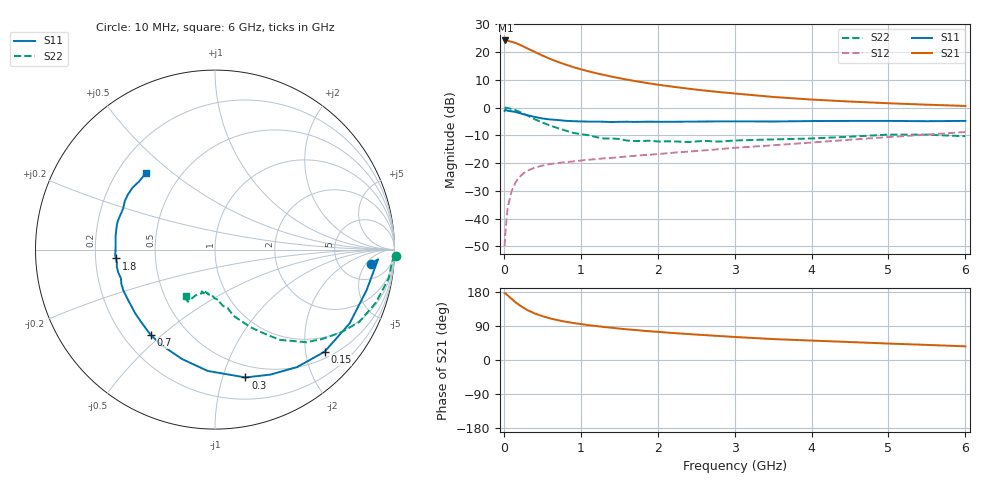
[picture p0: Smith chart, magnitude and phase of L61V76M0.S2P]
!  INFINEON TECHNOLOGIES Small Signal Semiconductors
! BFR380L3 , Si-NPN RF-Transistor in TSLP-3-1
!  Vce=1.75 V,  Ic=6 mA
! Common Emitter S-Parameters:  07. March 2005
#  GHz  S  MA  R  50
! f  S11  S21  S12  S22
! GHz  Mag  Ang  Mag  Ang  Mag  Ang  Mag  Ang
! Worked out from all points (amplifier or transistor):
!   36 points, 10 MHz to 6 GHz, reference 50 ohm
!   highest |S21| = 24.1 dB at 20 MHz (marker M1)
!   |S21| within 3 dB of that: start of sweep to 315.8 MHz
!   unconditionally stable (mu >= 1): 2.318 GHz to 4.796 GHz
!   at 250 MHz: K = 0.19, MSG = 22.9 dB, |S12| = -23.8 dB
!   at 1.4 GHz: K = 0.80, MSG = 14.6 dB, |S12| = -18.1 dB
!   at 6 GHz: K = 0.96, MSG = 4.7 dB, |S12| = -8.8 dB
!   S11 on the Smith chart (normalised r, x): 10 MHz: 10, -7; 150 MHz: 0.64, -2.39; 300 MHz: 0.39, -1.19; 700 MHz: 0.31, -0.46; 1.8 GHz: 0.29, -0.04; 6 GHz: 0.32, +0.41
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0.01  0.8704 -5.3  16.06 176.4  0.0032 83.3  1.01 -1.9
0.02  0.9101 -3.4  16.12 176.4  0.0056 87.8  0.9887 -3.8
0.05  0.8743 -15.0  15.87 170.4  0.0157 82.8  0.9813 -9.3
0.1  0.8554 -28.8  15.29 161.5  0.0311 76.1  0.9442 -18.2
0.15  0.8345 -43.0  14.59 152.8  0.0444 68.4  0.8992 -26.6
0.2  0.7984 -55.1  13.63 145.1  0.0554 63.7  0.8413 -33.2
0.25  0.7618 -66.1  12.67 138.6  0.0647 58.4  0.7771 -39.9
0.3  0.7323 -76.6  11.69 132.5  0.0721 54.4  0.7249 -45.4
0.4  0.6774 -93.4  10.05 122.9  0.0829 48.7  0.6181 -54.4
0.5  0.6367 -106.8  8.654 115.8  0.0903 45.7  0.5372 -60.0
0.6  0.6109 -118.2  7.517 109.8  0.0961 43.2  0.4765 -65.3
0.7  0.596 -126.8  6.651 105.2  0.1004 42.3  0.4264 -69.6
0.9  0.5689 -141.5  5.357 97.7  0.1072 41.5  0.3506 -76.6
1.1  0.5591 -151.2  4.49 92.0  0.1148 42.4  0.3177 -81.7
1.4  0.548 -162.9  3.599 85.2  0.1239 43.9  0.2777 -87.5
1.8  0.5542 -174.9  2.856 77.4  0.1387 46.9  0.2506 -95.0
2.2  0.5545 176.7  2.369 71.2  0.1539 49.9  0.2471 -99.8
2.8  0.5638 165.9  1.901 63.3  0.1782 53.8  0.2439 -107.6
3.5  0.5606 155.9  1.551 55.2  0.2092 55.8  0.267 -111.2
4.5  0.5739 147.8  1.282 47.4  0.2637 58.6  0.2989 -115.2
5.5  0.5683 138.1  1.125 39.8  0.3265 58.2  0.3248 -118.9
6  0.5747 132.1  1.069 36.1  0.362 56.9  0.3047 -121.7
